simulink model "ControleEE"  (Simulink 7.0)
settings: Solver=ode45  StartTime=0.0  StopTime=40  RelTol=1e-6
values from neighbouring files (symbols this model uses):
  K = acker(A,B,[p p])    [para2nl.m]    (also in para2nl_PI.m = acker(Aa,Ba,[p,p,p]); PrPara2nl_PI.m = acker(Aa,Ba,[p,p,p]); TestesEE.m = acker(A,B,[p,-.6-1.02i,-.6+1.02i]); TestesEEobsPert.m = acker(A,B,[p,-.6-1.0198i,-.6+1.0198i]))
  L = L'    [para2nl.m]    (also in para2nl_PI.m; PrPara2nl_PI.m; TestesEE.m; TestesEEcanalI.m)
  Nb = gf.den{1}(1,3)/gf.num{1}(1,3)    [para2nl.m]    (also in PrPara2nl_PI.m; TestesEE.m = gf.den{1}(1,4)/gf.num{1}(1,4); TestesEEcanalI.m = -Ki/(100*p); TestesEEobsPert.m = gf.den{1}(1,4)/gf.num{1}(1,4))

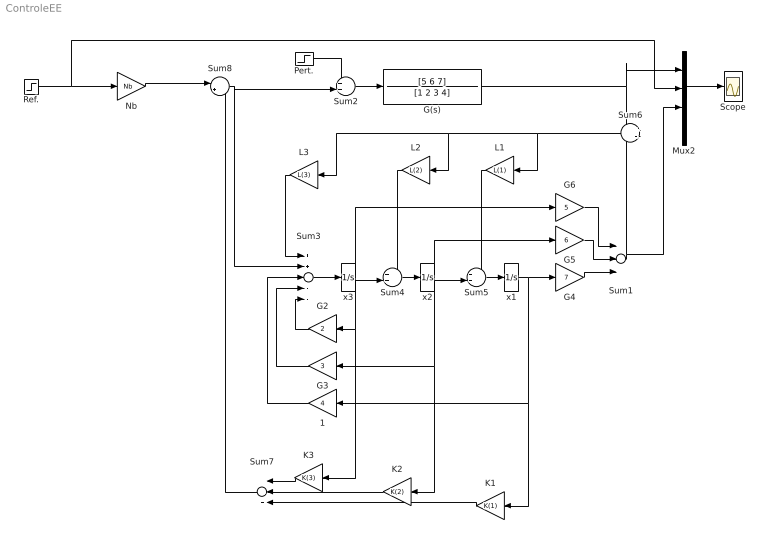
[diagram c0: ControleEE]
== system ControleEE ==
  1 : Gain  Orientation=left  Gain=4  ParameterDataType=sfix(16)  ParameterScaling=2^0  OutDataType=sfix(16)  OutScaling=2^0
  G(s) : TransferFcn  Numerator=[5 6 7]  Denominator=[1 2 3 4]
  G2 : Gain  Orientation=left  Gain=2  ParameterDataType=sfix(16)  ParameterScaling=2^0  OutDataType=sfix(16)  OutScaling=2^0
  G3 : Gain  Orientation=left  Gain=3  ParameterDataType=sfix(16)  ParameterScaling=2^0  OutDataType=sfix(16)  OutScaling=2^0
  G4 : Gain  Gain=7  ParameterDataType=sfix(16)  ParameterScaling=2^0  OutDataType=sfix(16)  OutScaling=2^0
  G5 : Gain  Gain=6  ParameterDataType=sfix(16)  ParameterScaling=2^0  OutDataType=sfix(16)  OutScaling=2^0
  G6 : Gain  Gain=5  ParameterDataType=sfix(16)  ParameterScaling=2^0  OutDataType=sfix(16)  OutScaling=2^0
  K1 : Gain  Orientation=left  Gain=K(1)  ParameterDataType=sfix(16)  ParameterScaling=2^0  OutDataType=sfix(16)  OutScaling=2^0
  K2 : Gain  Orientation=left  Gain=K(2)  ParameterDataType=sfix(16)  ParameterScaling=2^0  OutDataType=sfix(16)  OutScaling=2^0
  K3 : Gain  Orientation=left  Gain=K(3)  ParameterDataType=sfix(16)  ParameterScaling=2^0  OutDataType=sfix(16)  OutScaling=2^0
  L1 : Gain  Orientation=left  Gain=L(1)  ParameterDataType=sfix(16)  ParameterScaling=2^0  OutDataType=sfix(16)  OutScaling=2^0
  L2 : Gain  Orientation=left  Gain=L(2)  ParameterDataType=sfix(16)  ParameterScaling=2^0  OutDataType=sfix(16)  OutScaling=2^0
  L3 : Gain  Orientation=left  Gain=L(3)  ParameterDataType=sfix(16)  ParameterScaling=2^0  OutDataType=sfix(16)  OutScaling=2^0
  Mux2 : Mux
  Nb : Gain  Gain=Nb  ParameterDataType=sfix(16)  ParameterScaling=2^0  OutDataType=sfix(16)  OutScaling=2^0
  Pert. : Step  Time=10  SampleTime=0
  Ref. : Step  Time=5  SampleTime=0
  Scope : Scope
  Sum1 : Sum  Inputs=+++  OutDataType=sfix(16)  OutScaling=2^0
  Sum2 : Sum  Inputs=++|  OutDataType=sfix(16)  OutScaling=2^0
  Sum3 : Sum  Inputs=++---  OutDataType=sfix(16)  OutScaling=2^0
  Sum4 : Sum  Inputs=++|  OutDataType=sfix(16)  OutScaling=2^0
  Sum5 : Sum  Inputs=++|  OutDataType=sfix(16)  OutScaling=2^0
  Sum6 : Sum  Orientation=left  Inputs=+-  OutDataType=sfix(16)  OutScaling=2^0
  Sum7 : Sum  Orientation=left  Inputs=+++  OutDataType=sfix(16)  OutScaling=2^0
  Sum8 : Sum  Inputs=|+-  OutDataType=sfix(16)  OutScaling=2^0
  x1 : Integrator
  x2 : Integrator
  x3 : Integrator
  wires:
  Ref./1 -> Nb/1, Mux2/2
  Mux2/1 -> Scope/1
  x3/1 -> G6/1, Sum4/2, G2/1, K3/1
  x2/1 -> G5/1, Sum5/2, G3/1, K2/1
  Sum3/1 -> x3/1
  G2/1 -> Sum3/5
  G3/1 -> Sum3/4
  x1/1 -> G4/1, 1/1, K1/1
  1/1 -> Sum3/3
  G4/1 -> Sum1/3
  G5/1 -> Sum1/2
  G6/1 -> Sum1/1
  G(s)/1 -> Sum6/1, Mux2/1
  Sum1/1 -> Sum6/2, Mux2/3
  Sum2/1 -> G(s)/1
  Sum4/1 -> x2/1
  Sum5/1 -> x1/1
  L3/1 -> Sum3/1
  L2/1 -> Sum4/1
  L1/1 -> Sum5/1
  Pert./1 -> Sum2/1
  K3/1 -> Sum7/1
  K2/1 -> Sum7/2
  K1/1 -> Sum7/3
  Sum8/1 -> Sum3/2, Sum2/2
  Nb/1 -> Sum8/1
  Sum6/1 -> L3/1, L2/1, L1/1
  Sum7/1 -> Sum8/2
